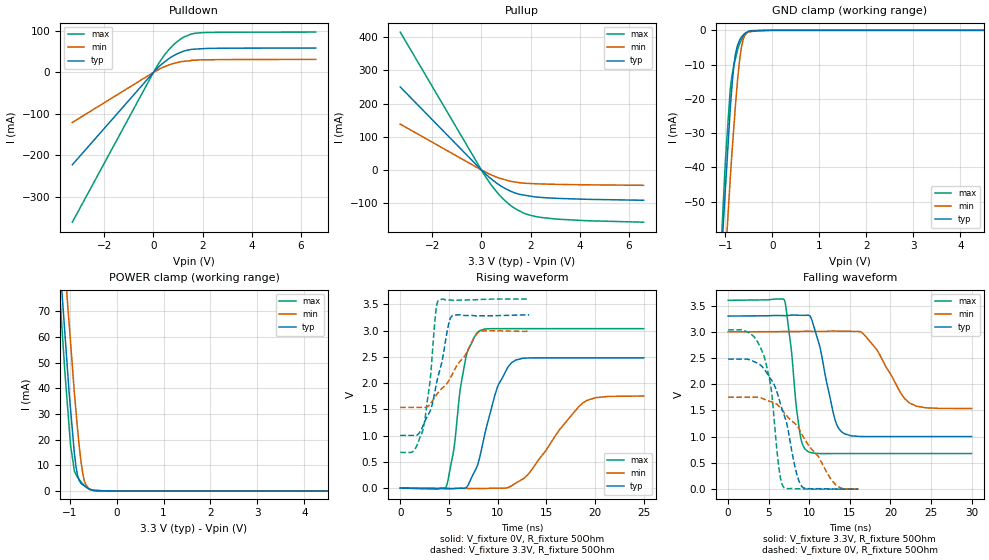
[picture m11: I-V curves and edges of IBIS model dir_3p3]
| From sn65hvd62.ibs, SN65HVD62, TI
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|   dir_3p3 Model
[Model]   dir_3p3
Model_type   3-state
Polarity   Non-Inverting
Vmeas = 1.65
Vref = 1.65
Cref = 2pF
Rref = 50
|   typ   min   max
|   (nom PVT)   (fast PVT)   (slow PVT)
 C_comp   2.476e-12   2.314e-12   2.799e-12
|ON state : BUFFER OUTPUT TURNED HIGH
|C_comp   2.476e-12   2.314e-12   2.799e-12
|OFF state: BUFFER IN HIGH IMPEDANCE
|C_comp   1.569e-12   1.546e-12   1.593e-12
| Where nom  PVT is Nominal Process, 3.3V, 27C
|   Fast PVT is Strong Process,  3.6V, -40C
|   Slow PVT is Weak Process,   3V, 125C
[Voltage Range]   3.3   3   3.6
|Ambient Temperature   25   85   -40
|Junction Temperature
[Temperature Range]   27   125   -40
[Pullup Reference]   3.3   3   3.6
[Pulldown Reference]   0   0   0
[Power Clamp Reference]   3.3   3   3.6
[GND Clamp Reference]   0   0   0
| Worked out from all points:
|   slope of the pulldown table from 0 to 0.495 V, typ, clamps not added: 18.1 ohm
|   slope of the pullup table from 0 to 0.495 V, typ, clamps not added: 15.2 ohm
|   GND clamp passes 1 mA (typ) near -0.60 V on its own axis
|   POWER clamp passes 1 mA (typ) near -0.61 V on its own axis
|   falling waveform, V_fixture 3.3V, R_fixture 50Ohm: 20-80 % time 1.88ns typ, 3.21ns min, 1.18ns max; typ from 3.3 V to 1 V
|   rising waveform, V_fixture 0V, R_fixture 50Ohm: 20-80 % time 2.1ns typ, 4.16ns min, 1.31ns max; typ from 0 V to 2.48 V
|   rising waveform, V_fixture 3.3V, R_fixture 50Ohm: 20-80 % time 1.62ns typ, 3.19ns min, 985ps max; typ from 1 V to 3.3 V
|   falling waveform, V_fixture 0V, R_fixture 50Ohm: 20-80 % time 2.45ns typ, 4.84ns min, 1.48ns max; typ from 2.48 V to 0 V
[Pulldown]
|   Voltage   I(typ)   I(min)   I(max)
-3.3V     -222.8mA   -120.8mA   -361.4mA
136.8mV   8.66mA     4.456mA    14.42mA
478.8mV   26.54mA    14.51mA    44.44mA
633.6mV   33.67mA    18.14mA    55.46mA
939.6mV   44.17mA    23.26mA    73.06mA
1.246V    51.43mA    26.71mA    85.55mA
1.534V    55.43mA    28.33mA    92.57mA
1.89V     56.88mA    30.22mA    95.56mA
6.6V      58.77mA    31.34mA    97.28mA
[GND Clamp]
|   Voltage   I(typ)   I(min)   I(max)
-3.3V     -755.7mA   -695.5mA   -833.4mA
-1.166V   -88.36mA   -104.7mA   -84.23mA
-1.049V   -57.66mA   -78.04mA   -51.76mA
-1.001V   -46.6mA    -66.97mA   -38.27mA
-896.4mV  -22.9mA    -43.21mA   -17.16mA
-854.7mV  -15.35mA   -34.83mA   -12.88mA
-785.4mV  -6.918mA   -21.81mA   -8.29mA
-702mV    -3.048mA   -9.283mA   -4.018mA
-660mV    -1.98mA    -5.059mA   -2.863mA
-591mV    -929.6uA   -1.573mA   -1.187mA
-501.6mV  -276.3uA   -484.8uA   -298.1uA
6.6V      0A         0A         0A
[Pullup]
|   Voltage   I(typ)   I(min)   I(max)
-3.3V     250.2mA    138.2mA    415.6mA
86.4mV    -6.262mA   -3.341mA   -10.56mA
342mV     -23.64mA   -13.01mA   -39.16mA
633.6mV   -40.52mA   -22.08mA   -67.07mA
1.123V    -61.74mA   -32.78mA   -103.2mA
1.364V    -69.15mA   -36.31mA   -116.2mA
1.706V    -75.49mA   -39.56mA   -129.6mA
2.012V    -79.28mA   -41.01mA   -137.2mA
2.473V    -83.05mA   -42.27mA   -143.5mA
4.162V    -88.17mA   -44.65mA   -152.6mA
6.6V      -91.37mA   -46.33mA   -157.5mA
[POWER Clamp]
|   Voltage   I(typ)   I(min)   I(max)
-3.3V     718.1mA    707.1mA    746.1mA
-1.206V   89.27mA    114.4mA    75.66mA
-1.178V   81.58mA    107.3mA    68.01mA
-1.094V   60.15mA    85.77mA    45.11mA
-1.01V    38.48mA    65.39mA    25.13mA
-979.2mV  31.98mA    58.02mA    17.9mA
-896.4mV  14.48mA    38.09mA    7.714mA
-864.6mV  9.677mA    31.31mA    6.547mA
-795.3mV  4.1mA      17.65mA    4.472mA
-723mV    2.433mA    7.259mA    2.811mA
-576mV    655.5uA    767.2uA    613.1uA
6.6V      0A         0A         0A
[Ramp]
R_load = 50
|   typ   min   max
dV/dt_r   1.48829/2.09663e-09   1.05218/4.15612e-09   1.82234/1.30144e-09
dV/dt_f   1.37807/1.88167e-09   0.877328/3.20296e-09   1.75255/1.17455e-09
[Falling Waveform]
V_fixture = 3.3V
V_fixture_min = 3V
V_fixture_max = 3.6V
R_fixture = 50Ohm
|   Time   V(typ)   V(min)   V(max)
0s        3.3V       3V         3.6V
6.914ns   3.309V     3.006V     3.61V
8.807ns   3.315V     3.005V     1.104V
9.77ns    3.316V     3.01V      723.4mV
11.24ns   2.75V      3.007V     678.9mV
13.16ns   1.327V     3.014V     678.8mV
13.96ns   1.095V     3.011V     679mV
16.79ns   1.003V     2.94V      679.1mV
22.34ns   1.003V     1.644V     679.1mV
30ns      1.003V     1.538V     679.1mV
[Rising Waveform]
V_fixture = 0V
V_fixture_min = 0V
V_fixture_max = 0V
R_fixture = 50Ohm
|   Time   V(typ)   V(min)   V(max)
0s        4.047nV    27.6nV     2.807nV
4.709ns   -11.71mV   -3.241mV   20.11mV
5.492ns   -11.05mV   -6.103mV   726.5mV
6.137ns   -538.8uV   -5.706mV   1.85V
6.749ns   7.321mV    -5.553mV   2.493V
8.153ns   579.1mV    -8.151mV   2.995V
9.971ns   1.919V     -352.4uV   3.037V
11.85ns   2.437V     95.19mV    3.037V
18.73ns   2.48V      1.619V     3.037V
25ns      2.48V      1.754V     3.037V
[Rising Waveform]
V_fixture = 3.3V
V_fixture_min = 3V
V_fixture_max = 3.6V
R_fixture = 50Ohm
|   Time   V(typ)   V(min)   V(max)
0s        1.003V     1.538V     679.1mV
1.343ns   1.003V     1.538V     702.8mV
2.366ns   1.199V     1.537V     1.13V
3.059ns   1.462V     1.597V     2.029V
3.608ns   1.885V     1.746V     3.283V
3.896ns   2.135V     1.82V      3.569V
4.976ns   3.128V     2.04V      3.581V
5.348ns   3.285V     2.17V      3.581V
8.27ns    3.282V     2.991V     3.592V
13.24ns   3.3V       2.988V     3.6V
[Falling Waveform]
V_fixture = 0V
V_fixture_min = 0V
V_fixture_max = 0V
R_fixture = 50Ohm
|   Time   V(typ)   V(min)   V(max)
0s        2.48V      1.754V     3.037V
2.744ns   2.462V     1.754V     2.966V
4.412ns   2.297V     1.717V     2.54V
5.318ns   2.084V     1.665V     1.893V
6.347ns   1.678V     1.567V     301.7mV
6.899ns   1.41V      1.459V     26.32mV
8.282ns   392.6mV    1.245V     6.937mV
9.074ns   50.68mV    1.05V      4.762mV
13.27ns   2.367mV    79.77mV    -7.009uV
16.05ns   4.689uV    4.615mV    294.4nV
